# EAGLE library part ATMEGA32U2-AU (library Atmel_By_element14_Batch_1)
8-bit Microcontroller with ISP Flash and USB Controller
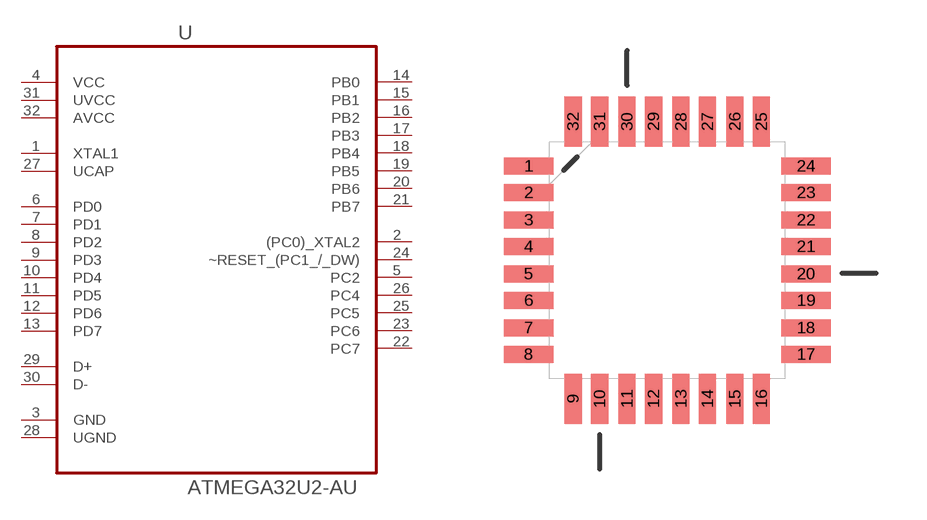
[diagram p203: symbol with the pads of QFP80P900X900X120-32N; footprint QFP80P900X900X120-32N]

Designator prefix U

## ATMEGA32U2-AU (MPN: ATMEGA32U2-AU; OC_FARNELL: 1748524; OC_NEWARK: 26R5632; PACKAGE: TQFP-32; SUPPLIER: Atmel)  [QFP80P900X900X120-32N]
1  XTAL1  in
2  (PC0)_XTAL2
3  GND  pas
4  VCC  pwr
5  PC2
6  PD0
7  PD1
8  PD2
9  PD3
10  PD4
11  PD5
12  PD6
13  PD7
14  PB0
15  PB1
16  PB2
17  PB3
18  PB4
19  PB5
20  PB6
21  PB7
22  PC7
23  PC6
24  ~RESET_(PC1_/_DW)
25  PC5
26  PC4
27  UCAP  pwr
28  UGND  pas
29  D+
30  D-
31  UVCC  pwr
32  AVCC  pwr

## Footprint QFP80P900X900X120-32N (pad centres in mm)
smd 1.473 x 0.508: 1 -4.115,2.794; 2 -4.115,2.007; 3 -4.115,1.194; 4 -4.115,0.406; 5 -4.115,-0.406; 6 -4.115,-1.194; 7 -4.115,-2.007; 8 -4.115,-2.794; 17 4.115,-2.794; 18 4.115,-2.007; 19 4.115,-1.194; 20 4.115,-0.406; 21 4.115,0.406; 22 4.115,1.194; 23 4.115,2.007; 24 4.115,2.794
smd 0.508 x 1.473: 9 -2.794,-4.115; 10 -2.007,-4.115; 11 -1.194,-4.115; 12 -0.406,-4.115; 13 0.406,-4.115; 14 1.194,-4.115; 15 2.007,-4.115; 16 2.794,-4.115; 25 2.794,4.115; 26 2.007,4.115; 27 1.194,4.115; 28 0.406,4.115; 29 -0.406,4.115; 30 -1.194,4.115; 31 -2.007,4.115; 32 -2.794,4.115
